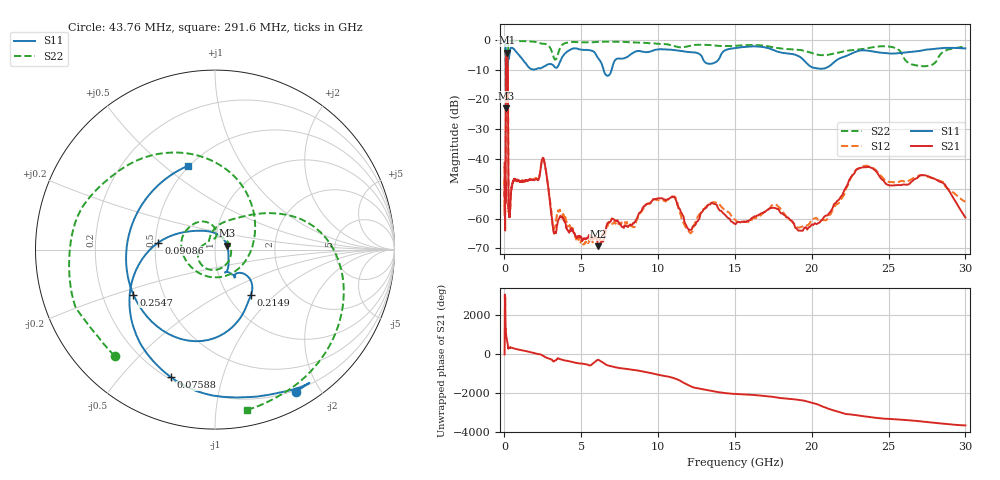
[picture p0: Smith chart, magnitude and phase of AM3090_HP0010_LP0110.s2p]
! Date/Time: Thu, Feb 28, 2019 1:55 PM
! Network Analyzer: Agilent Technologies E8364B Rev: A.07.50.67
! Sweep from 0.010 to 30.000 GHz, 1601 Points, Sweep Type: LOG
! Power Supply: 5.023 V, 0.002 A
# Hz S DB R 50
!freq MagS11 AngS11 MagS21 AngS21 MagS12 AngS12 MagS22 AngS22
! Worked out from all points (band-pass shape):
!   1601 points, 10 MHz to 30 GHz, reference 50 ohm
!   highest |S21| = -4.29 dB at 148.4 MHz (marker M1); lowest = -69.3 dB at 6.11 GHz (marker M2)
!   |S21| within 3 dB of the highest: 101.3 MHz to 210.5 MHz (109.2 MHz wide, 70 % of centre)
!   lowest |S11| = -22.9 dB at 99.43 MHz (marker M3), VSWR 1.15, Z = 57.2 + j2.55 ohm
!   |S11| at or under -10 dB: 90.88 MHz to 213.4 MHz (122.5 MHz wide, 80.5 % of centre); 6.451 GHz to 6.979 GHz (527.6 MHz wide, 7.86 % of centre)
!   |S22| runs from -25.1 to -0.2 dB; largest |S21 - S12| = 0.012
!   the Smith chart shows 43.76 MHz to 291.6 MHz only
!   S11 on the Smith chart (normalised r, x): 43.76 MHz: 0.18, -1.71; 75.88 MHz: 0.21, -0.69; 90.86 MHz: 0.52, +0.05; 214.9 MHz: 1.27, -0.72; 254.7 MHz: 0.34, -0.23; 291.6 MHz: 0.49, +0.60
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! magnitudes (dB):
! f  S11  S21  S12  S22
! 10 MHz  -0.3  -41.3  -42.8  -0.6
! 38.04 MHz  -0.5  -60.8  -60.7  -1.4
! 43.76 MHz  -0.8  -60.6  -61.7  -1.8
! 48.61 MHz  -0.8  -50.8  -48.1  -1.6
! 75.88 MHz  -2.5  -47.7  -47.5  -4.5
! 90.86 MHz  -10.0  -15.9  -15.8  -16.0
! 99.43 MHz  -22.9  -8.0  -8.0  -14.2
! 144.7 MHz  -15.4  -4.3  -4.3  -21.5
! 148.4 MHz  -15.3  -4.3  -4.3  -21.0
! 214.9 MHz  -9.8  -8.2  -8.2  -15.3
! 254.7 MHz  -5.7  -49.9  -48.0  -1.9
! 291.6 MHz  -6.2  -57.3  -56.1  -0.8
! 550.5 MHz  -2.8  -47.6  -47.9  -0.3
! 2.084 GHz  -9.8  -46.6  -46.5  -0.7
! 2.533 GHz  -9.0  -39.7  -39.8  -1.3
! 3.253 GHz  -9.0  -64.9  -63.0  -6.4
! 6.11 GHz  -6.2  -69.3  -66.6  -0.6
! 7.926 GHz  -5.9  -62.5  -61.6  -0.7
! 10.65 GHz  -3.3  -53.4  -53.7  -1.5
! 19.7 GHz  -8.0  -63.7  -62.3  -3.9
! 23.48 GHz  -3.5  -42.8  -42.3  -2.9
! 30 GHz  -2.8  -59.7  -54.3  -2.3
